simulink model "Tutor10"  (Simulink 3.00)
settings: Solver=ode45  SolverMode=SingleTasking  StartTime=0.0  StopTime=10  RelTol=1e-3  AbsTol=1e-3
libraries: simulink3 x1

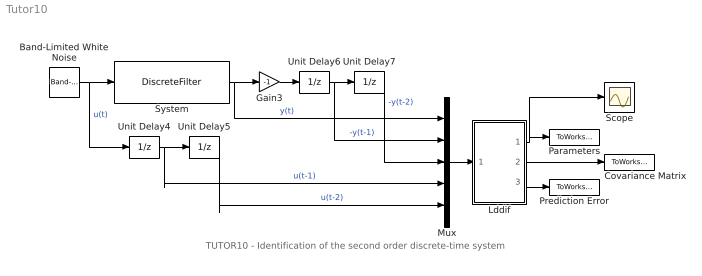
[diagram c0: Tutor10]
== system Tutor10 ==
  note: TUTOR10 - Identification of the second order discrete-time system
  Band-Limited White Noise : simulink3/Sources/Band-Limited White Noise  Cov=[0.1]  Ts=0.1  seed=[23341]
  Covariance Matrix : ToWorkspace  VariableName=CovMatrix  SampleTime=0  SaveFormat=Matrix
  Gain3 : Gain  Gain=-1  SaturateOnIntegerOverflow=on
  Lddif : Subsystem  mask(LDDIF){par=[4,1], L=[0.985], d=[0.01], poc=[0 0 0 0], kov=[10e6], ts=[1]}
      mask prompts: par "No. of estimated parameters and outputs - [n,m]:"; L "Exponential forgetting - [L]:"; d "Bittanti's correction - [d]:"; poc "Initial parameter estimates - [theta(1) ... theta(n)]:"; kov "Covariance matrix (see help, standard - [10e6]):"; ts "Sampling period - [ts]:"
      mask help: LDDIF: + Bittanti's corrections Authors: Lubos Cirka and Miroslav Fikar 1998 - 2004
      mask init:
      | n=par(1); m=par(2);
  Mux : Mux  Inputs=5
  Parameters : ToWorkspace  VariableName=BA  SampleTime=0  SaveFormat=Matrix
  Prediction Error : ToWorkspace  VariableName=PredError  SampleTime=0  SaveFormat=Matrix
  Scope : Scope
  System : DiscreteFilter  Numerator=[0 0.8 0.2]  Denominator=[1 -0.5 0.06]  SampleTime=1
  Unit Delay{4..7} (4 alike) : UnitDelay  X0=0  SampleTime=1
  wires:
  System/1 -> Mux/1, Gain3/1  "y(t)"
  Unit Delay6/1 -> Mux/2, Unit Delay7/1  "-y(t-1)"
  Gain3/1 -> Unit Delay6/1
  Unit Delay4/1 -> Mux/4, Unit Delay5/1  "u(t-1)"
  Band-Limited White Noise/1 -> Unit Delay4/1, System/1  "u(t)"
  Mux/1 -> Lddif/1("y, z")
  Unit Delay7/1 -> Mux/3  "-y(t-2)"
  Unit Delay5/1 -> Mux/5  "u(t-2)"
  Lddif/2(covariance matrix) -> Covariance Matrix/1
  Lddif/3(prediction error) -> Prediction Error/1
  Lddif/1(theta) -> Parameters/1, Scope/1

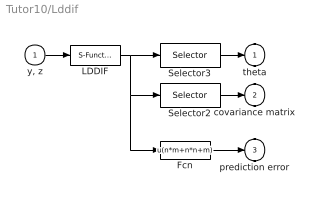
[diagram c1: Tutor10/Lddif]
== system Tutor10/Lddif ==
  "y, z" : Inport  Port=1  PortWidth=-1  SampleTime=-1  DataType=auto
  Fcn : Fcn  Expr=u(n*m+n*n+m)
  LDDIF : S-Function  FunctionName=lddif_s  Parameters=m, n, L, d, poc, kov, ts  PortCounts=[]  SFunctionModules=''
  Selector2 : Selector  Elements=[n*m:1:n*m+n*n]  InputPortWidth=n*m+n*n+m
  Selector3 : Selector  Elements=[1:1:n*m]  InputPortWidth=n*m+n*n+m
  theta : Outport  Port=1  InitialOutput=0
  covariance matrix : Outport  Port=2  InitialOutput=0
  prediction error : Outport  Port=3  InitialOutput=0
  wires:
  "y, z"/1 -> LDDIF/1
  LDDIF/1 -> Selector3/1, Selector2/1, Fcn/1
  Selector2/1 -> covariance matrix/1
  Selector3/1 -> theta/1
  Fcn/1 -> prediction error/1
